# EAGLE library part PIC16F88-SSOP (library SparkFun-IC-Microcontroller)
8-Bit PIC16F8X Family Pin Compatible : PIC16F83, PIC16CR83, PIC16F84A, PIC16CR84 RETIRED
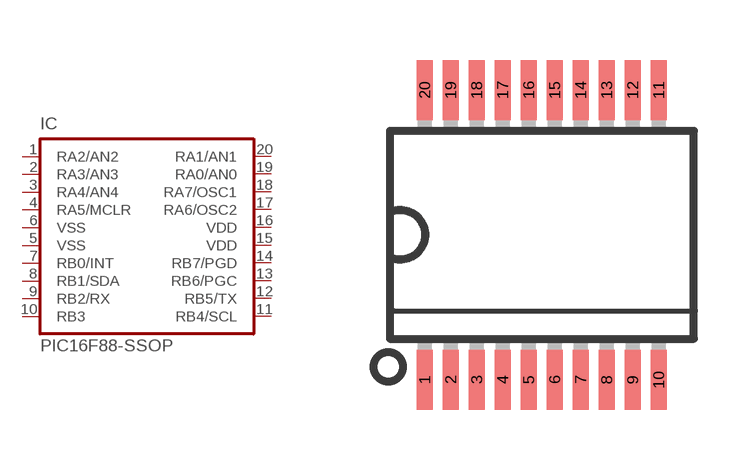
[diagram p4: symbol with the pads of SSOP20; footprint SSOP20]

Designator prefix IC

## PIC16F88-SSOP  [SSOP20]
1  RA2/AN2
2  RA3/AN3
3  RA4/AN4
4  RA5/MCLR  in
5  VSS  pwr
6  VSS  pwr
7  RB0/INT
8  RB1/SDA
9  RB2/RX
10  RB3
11  RB4/SCL
12  RB5/TX
13  RB6/PGC
14  RB7/PGD
15  VDD  pwr
16  VDD  pwr
17  RA6/OSC2
18  RA7/OSC1
19  RA0/AN0
20  RA1/AN1

## Footprint SSOP20 (pad centres in mm)
Shrink Small Outline Package package type SS
smd 0.4 x 1.5: 1 -2.925,-3.625; 2 -2.275,-3.625; 3 -1.625,-3.625; 4 -0.975,-3.625; 5 -0.325,-3.625; 6 0.325,-3.625; 7 0.975,-3.625; 8 1.625,-3.625; 9 2.275,-3.625; 10 2.925,-3.625; 11 2.925,3.625; 12 2.275,3.625; 13 1.625,3.625; 14 0.975,3.625; 15 0.325,3.625; 16 -0.325,3.625; 17 -0.975,3.625; 18 -1.625,3.625; 19 -2.275,3.625; 20 -2.925,3.625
